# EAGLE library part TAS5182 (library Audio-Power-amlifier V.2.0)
100−W STEREO DIGITAL AMPLIFIER POWER STAGE CONTROLLER
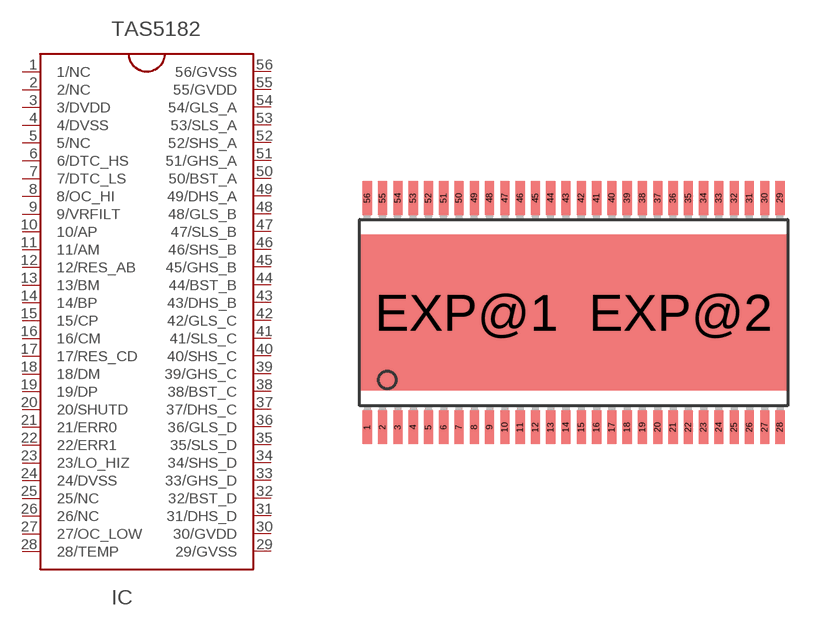
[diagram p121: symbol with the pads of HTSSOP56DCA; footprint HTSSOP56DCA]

Designator prefix IC

## TAS5182  [HTSSOP56DCA]
1  1/NC  nc
2  2/NC  nc
3  3/DVDD  pwr
4  4/DVSS  pwr
5  5/NC  nc
6  6/DTC_HS  in
7  7/DTC_LS  in
8  8/OC_HI  in
9  9/VRFILT  in
10  10/AP  in
11  11/AM  in
12  12/RES_AB  in
13  13/BM  in
14  14/BP  in
15  15/CP  in
16  16/CM  in
17  17/RES_CD  in
18  18/DM  in
19  19/DP  in
20  20/SHUTD  out
21  21/ERR0  out
22  22/ERR1  out
23  23/LO_HIZ  in
24  24/DVSS  pwr
25  25/NC  nc
26  26/NC  nc
27  27/OC_LOW  in
28  28/TEMP  in
29  29/GVSS  pwr
30  30/GVDD  pwr
31  31/DHS_D  in
32  32/BST_D  in
33  33/GHS_D  out
34  34/SHS_D  in
35  35/SLS_D  in
36  36/GLS_D  out
37  37/DHS_C  in
38  38/BST_C  in
39  39/GHS_C  out
40  40/SHS_C  in
41  41/SLS_C  in
42  42/GLS_C  out
43  43/DHS_B  in
44  44/BST_B  in
45  45/GHS_B  out
46  46/SHS_B  in
47  47/SLS_B  in
48  48/GLS_B  out
49  49/DHS_A  in
50  50/BST_A  in
51  51/GHS_A  out
52  52/SHS_A  in
53  53/SLS_A  in
54  54/GLS_A  out
55  55/GVDD  pwr
56  56/GVSS  pwr

## Footprint HTSSOP56DCA (pad centres in mm)
PowerPAD(TM) PLASTIC SMALL-OUTLINE PACKAGE DCA (R-PDSO-G**) Source: http://focus.ti.com/lit/ml/mpds044/mpds044.pdf / slma002.pdf
smd 0.3 x 1.1: 1 -6.75,-3.75; 2 -6.25,-3.75; 3 -5.75,-3.75; 4 -5.25,-3.75; 5 -4.75,-3.75; 6 -4.25,-3.75; 7 -3.75,-3.75; 8 -3.25,-3.75; 9 -2.75,-3.75; 10 -2.25,-3.75; 11 -1.75,-3.75; 12 -1.25,-3.75; 13 -0.75,-3.75; 14 -0.25,-3.75; 15 0.25,-3.75; 16 0.75,-3.75; 17 1.25,-3.75; 18 1.75,-3.75; 19 2.25,-3.75; 20 2.75,-3.75; 21 3.25,-3.75; 22 3.75,-3.75; 23 4.25,-3.75; 24 4.75,-3.75; 25 5.25,-3.75; 26 5.75,-3.75; 27 6.25,-3.75; 28 6.75,-3.75; 29 6.75,3.75; 30 6.25,3.75; 31 5.75,3.75; 32 5.25,3.75; 33 4.75,3.75; 34 4.25,3.75; 35 3.75,3.75; 36 3.25,3.75; 37 2.75,3.75; 38 2.25,3.75; 39 1.75,3.75; 40 1.25,3.75; 41 0.75,3.75; 42 0.25,3.75; 43 -0.25,3.75; 44 -0.75,3.75; 45 -1.25,3.75; 46 -1.75,3.75; 47 -2.25,3.75; 48 -2.75,3.75; 49 -3.25,3.75; 50 -3.75,3.75; 51 -4.25,3.75; 52 -4.75,3.75; 53 -5.25,3.75; 54 -5.75,3.75; 55 -6.25,3.75; 56 -6.75,3.75
smd 7 x 5.1: EXP@1 -3.5,0; EXP@2 3.5,0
